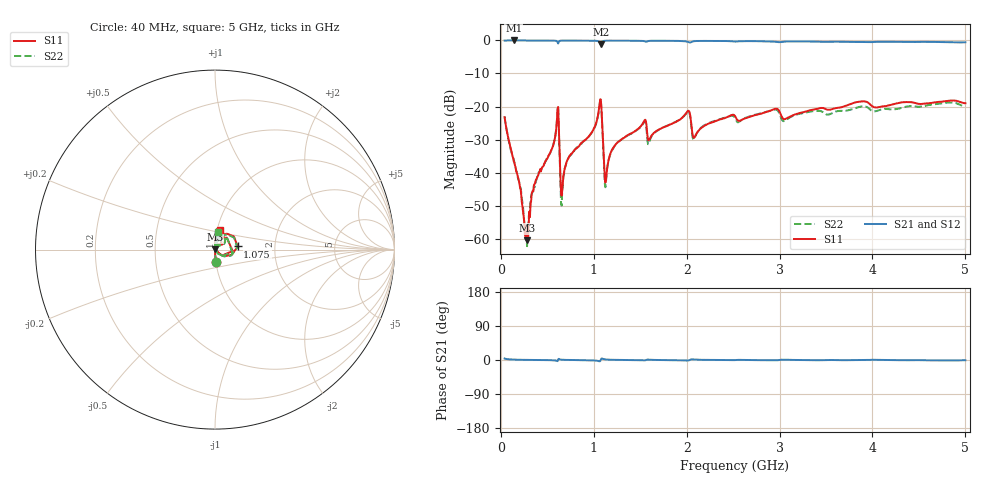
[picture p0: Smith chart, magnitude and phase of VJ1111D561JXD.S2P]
! VJ1111D561JXD
! DATE 02/15/2022  13:47
! CAPACITORS MOUNTED IN SERIES ON 25 MIL THICK MICROSTRIP SUBSTRATE
# GHz  S  MA  R  50.00
!  FREQ  S11M  S11A  S21M  S21A  S12M  S12A  S22M  S22A
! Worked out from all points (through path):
!   801 points, 40 MHz to 5 GHz, reference 50 ohm
!   highest |S21| = 0.00 dB at 139.2 MHz (marker M1); lowest = -1.2 dB at 1.075 GHz (marker M2)
!   lowest |S11| = -60.5 dB at 281.8 MHz (marker M3), VSWR 1.00, Z = 50.1 + j0.0607 ohm
!   |S11| at or under -10 dB: start of sweep to end of sweep
!   |S22| runs from -62.3 to -18.0 dB; largest |S21 - S12| = 0.011
!   S11 on the Smith chart (normalised r, x): 40 MHz: 1.00, -0.14; 1.075 GHz: 1.29, +0.05; 5 GHz: 1.03, +0.23
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0.04  0.0687 -84.0  0.998 3.9  0.9985 4.0  0.07096 -84.5
0.1392  0.0146 -86.7  1 1.0  0.9979 1.2  0.01575 -85.7
0.2818  0.0009433 40.0  0.9978 0.3  1 0.3  0.0007678 31.9
0.3562  0.00645 81.3  0.9966 0.1  1.001 0.1  0.006518 76.7
0.5484  0.02259 84.7  0.9941 -0.5  0.9995 -0.4  0.02263 84.0
0.598  0.04977 75.7  0.983 -1.9  0.9888 -1.9  0.04955 72.3
0.6662  0.006793 67.6  0.9957 0.6  0.9979 0.4  0.006489 76.0
0.722  0.0161 83.9  0.9951 0.1  0.9991 0.1  0.01612 84.4
0.8708  0.02822 86.1  0.9941 -0.3  0.9987 -0.3  0.0278 86.0
1.0754  0.1276 7.8  0.8709 0.9  0.8731 0.9  0.1246 5.1
1.1126  0.01205 -28.6  0.9865 2.0  0.9896 1.9  0.01053 -33.6
1.1374  0.009673 62.6  0.9914 1.2  0.9955 1.1  0.009404 66.6
1.2676  0.02935 87.8  0.9926 0.2  0.997 0.2  0.0294 86.0
1.5404  0.05969 76.8  0.9778 -0.9  0.9812 -1.0  0.05772 71.1
1.5962  0.03123 72.0  0.9841 0.8  0.9881 0.7  0.02881 75.2
1.6954  0.04418 87.1  0.9891 0.0  0.9939 -0.1  0.04441 86.0
2.0054  0.08324 71.1  0.959 -1.4  0.9649 -1.5  0.08177 66.5
2.086  0.0345 69.9  0.9775 1.3  0.9823 1.2  0.03369 71.0
2.52  0.0719 74.8  0.9627 -0.2  0.9694 -0.3  0.06697 72.0
3.3508  0.08918 86.1  0.9642 -0.4  0.9699 -0.6  0.08452 85.0
4.1754  0.104 81.9  0.9563 -0.3  0.9634 -0.4  0.09089 85.2
5  0.1119 76.3  0.9388 -0.6  0.945 -0.9  0.1016 80.1
